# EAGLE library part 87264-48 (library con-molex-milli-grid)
RECEPTACAL
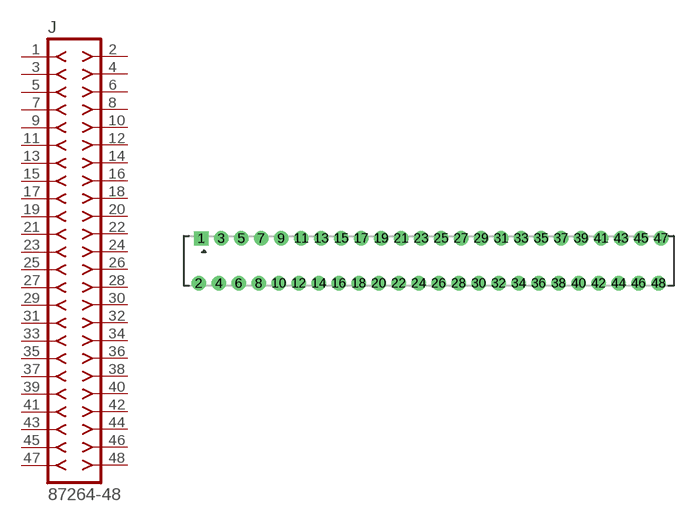
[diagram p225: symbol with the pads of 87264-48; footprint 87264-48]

Designator prefix J

## 87264-48  [87264-48]
1  1  pas
2  2  pas
3  3  pas
4  4  pas
5  5  pas
6  6  pas
7  7  pas
8  8  pas
9  9  pas
10  10  pas
11  11  pas
12  12  pas
13  13  pas
14  14  pas
15  15  pas
16  16  pas
17  17  pas
18  18  pas
19  19  pas
20  20  pas
21  21  pas
22  22  pas
23  23  pas
24  24  pas
25  25  pas
26  26  pas
27  27  pas
28  28  pas
29  29  pas
30  30  pas
31  31  pas
32  32  pas
33  33  pas
34  34  pas
35  35  pas
36  36  pas
37  37  pas
38  38  pas
39  39  pas
40  40  pas
41  41  pas
42  42  pas
43  43  pas
44  44  pas
45  45  pas
46  46  pas
47  47  pas
48  48  pas

## Footprint 87264-48 (pad centres in mm)
RECEPTACAL Dual Row, Side Entry
drill 0.914 square: 1 -22.75,2.25
drill 0.914: 2 -23,-2.25; 3 -20.75,2.25; 4 -21,-2.25; 5 -18.75,2.25; 6 -19,-2.25; 7 -16.75,2.25; 8 -17,-2.25; 9 -14.75,2.25; 10 -15,-2.25; 11 -12.75,2.25; 12 -13,-2.25; 13 -10.75,2.25; 14 -11,-2.25; 15 -8.75,2.25; 16 -9,-2.25; 17 -6.75,2.25; 18 -7,-2.25; 19 -4.75,2.25; 20 -5,-2.25; 21 -2.75,2.25; 22 -3,-2.25; 23 -0.75,2.25; 24 -1,-2.25; 25 1.25,2.25; 26 1,-2.25; 27 3.25,2.25; 28 3,-2.25; 29 5.25,2.25; 30 5,-2.25; 31 7.25,2.25; 32 7,-2.25; 33 9.25,2.25; 34 9,-2.25; 35 11.25,2.25; 36 11,-2.25; 37 13.25,2.25; 38 13,-2.25; 39 15.25,2.25; 40 15,-2.25; 41 17.25,2.25; 42 17,-2.25; 43 19.25,2.25; 44 19,-2.25; 45 21.25,2.25; 46 21,-2.25; 47 23.25,2.25; 48 23,-2.25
